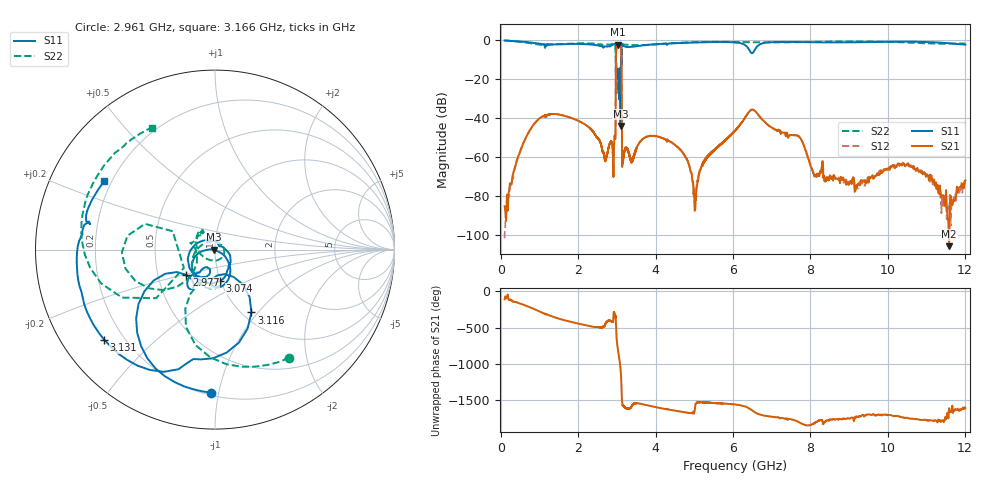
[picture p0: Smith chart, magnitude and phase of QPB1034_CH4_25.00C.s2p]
! TDS: k:\Engsetup\Winsaw\QPB1034_ALL
! Channel 1
! Ports=1 2
! seg 1=100.000000 1100.000000 51
! seg 2=1101.000000 1301.000000 201
! seg 3=1302.000000 2302.000000 101
! seg 4=2303.000000 3503.000000 1201
! seg 5=3504.000000 5204.000000 171
! seg 6=5205.000000 6405.000000 1201
! seg 7=6406.000000 8506.000000 211
! seg 8=8507.000000 12007.000000 176
! Points=3313
! FailCode=0
! Topology=ALL_SE(12)
!VNA Cal loaded =QPB1034_ALL_25C
!PS1(V)= 5.000
!PS(mA)= 0.432
!PS2(V)= 1.170
!PS(mA)= -0.001
!PS3(V)= 0.630
!PS(mA)= -0.001
!PS4(V)= 0.630
!PS(mA)= -0.002
!Temp (C)= 25.00
# MHz S DB R 50
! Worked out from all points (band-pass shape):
!   3313 points, 100 MHz to 12.01 GHz, reference 50 ohm
!   highest |S21| = -2.46 dB at 3.027 GHz (marker M1); lowest = -105.9 dB at 11.59 GHz (marker M2)
!   |S21| within 3 dB of the highest: 2.984 GHz to 3.114 GHz (130.4 MHz wide, 4.28 % of centre)
!   lowest |S11| = -44.2 dB at 3.095 GHz (marker M3), VSWR 1.01, Z = 49.4 - j0.092 ohm
!   |S11| at or under -10 dB: 2.975 GHz to 3.115 GHz (140 MHz wide, 4.6 % of centre)
!   |S22| runs from -27.3 to -0.3 dB; largest |S21 - S12| = 0.0042
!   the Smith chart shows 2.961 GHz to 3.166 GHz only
!   S11 on the Smith chart (normalised r, x): 2.961 GHz: 0.22, -0.95; 2.977 GHz: 0.70, -0.21; 3.074 GHz: 0.99, -0.36; 3.116 GHz: 1.10, -0.92; 3.131 GHz: 0.13, -0.35; 3.166 GHz: 0.17, +0.28
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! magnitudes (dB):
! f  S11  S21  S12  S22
! 100 MHz  -0.3  -85.4  -101.8  -0.3
! 240 MHz  -0.5  -73.5  -75.6  -0.5
! 500 MHz  -0.8  -57.4  -57.2  -0.9
! 1.1 GHz  -2.2  -39.1  -39.1  -2.6
! 2.434 GHz  -2.5  -48.5  -48.5  -1.9
! 2.908 GHz  -2.4  -67.4  -67.1  -2.1
! 2.961 GHz  -2.0  -50.9  -50.7  -2.7
! 2.977 GHz  -13.4  -9.9  -9.9  -14.9
! 3.027 GHz  -15.3  -2.5  -2.5  -19.6
! 3.074 GHz  -15.0  -3.0  -2.9  -18.1
! 3.095 GHz  -44.2  -3.2  -3.2  -18.5
! 3.116 GHz  -7.9  -6.5  -6.5  -7.4
! 3.131 GHz  -2.0  -47.6  -47.6  -2.4
! 3.146 GHz  -2.3  -61.2  -61.0  -2.2
! 3.166 GHz  -2.8  -61.9  -61.4  -2.3
! 4.084 GHz  -2.1  -49.8  -49.7  -2.2
! 5.034 GHz  -1.3  -81.2  -83.0  -1.2
! 5.406 GHz  -1.2  -58.7  -58.5  -1.0
! 6.496 GHz  -6.8  -35.8  -35.8  -1.2
! 8.496 GHz  -1.3  -70.4  -70.9  -0.9
! 11.59 GHz  -1.7  -105.9  -86.8  -2.0
! 12.01 GHz  -2.5  -72.2  -71.7  -1.8
